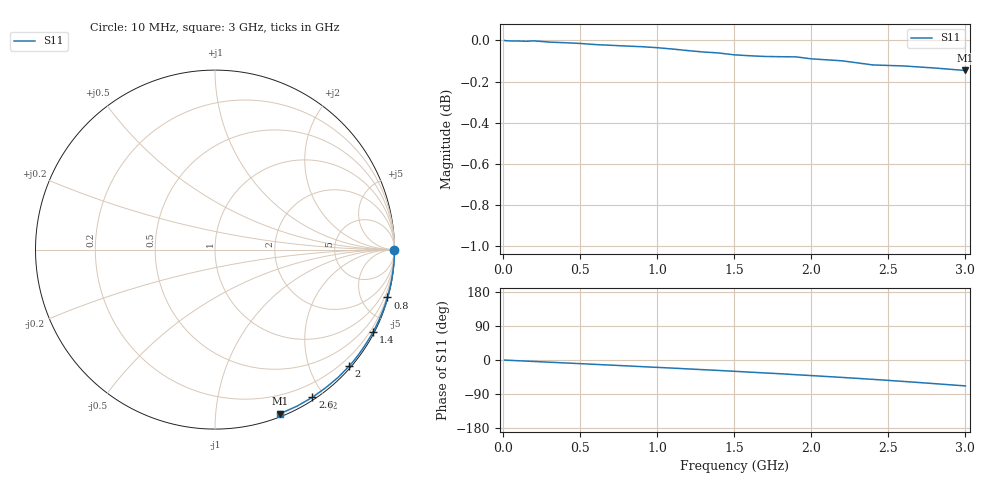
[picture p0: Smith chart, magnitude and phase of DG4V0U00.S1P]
! SIEMENS Small Signal Semiconductors
! BAV70
! Silicon Switching Diode in SOT23
! VR = 4 V
! S-Parameters:  May  1995
# GHz  S  MA  R  50
!  f  S11
! GHz  MAG  ANG
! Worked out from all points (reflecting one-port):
!   30 points, 10 MHz to 3 GHz, reference 50 ohm
!   lowest |S11| = -0.1 dB at 3 GHz (marker M1), VSWR 118.90, Z = 1.33 - j73.6 ohm
!   phase of S11 starts at -0 deg and turns -68 deg over the sweep
!   S11 on the Smith chart (normalised r, x): 10 MHz: open; 800 MHz: 0.09, -7.35; 1.4 GHz: 0.06, -4.07; 2 GHz: 0.04, -2.67; 2.6 GHz: 0.03, -1.86; 3 GHz: 0.03, -1.47
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0.01  1 -0.2
0.1  0.9997 -2.0
0.15  0.9995 -2.9
0.2  0.9998 -3.9
0.25  0.9994 -4.8
0.3  0.9991 -5.8
0.4  0.9987 -7.7
0.5  0.9983 -9.6
0.6  0.9977 -11.6
0.7  0.9973 -13.5
0.8  0.9969 -15.5
0.9  0.9965 -17.5
1  0.996 -19.5
1.1  0.9952 -21.4
1.2  0.9943 -23.5
1.3  0.9936 -25.6
1.4  0.993 -27.6
1.5  0.992 -29.8
1.6  0.9915 -32.0
1.7  0.9911 -34.2
1.8  0.9909 -36.3
1.9  0.9909 -38.8
2  0.9898 -41.1
2.2  0.9887 -46.0
2.4  0.9864 -51.1
2.6  0.9858 -56.6
2.8  0.9847 -62.4
3  0.9833 -68.4
